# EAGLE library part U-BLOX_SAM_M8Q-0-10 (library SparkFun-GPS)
u-blox SAM-M8Q The u-blox concurrent SAM-M8Q GNSS patch antenna module benefits from the exceptional performance of the u-blox M8 multi-GNSS engine. The SAM-M8Q module offers high sensitivity and minimal acquisition times in an ultra compact form factor. The SAM-M8Q module utilizes concurrent reception of up to three GNSS systems (GPS/Galileo and GLONASS), recognizes multiple constellations simultaneously and provides outstanding positioning accuracy in scenarios where urban canyon or weak signals are involved. For even better and faster positioning improvement, the SAM-M8Q supports augmentation of QZSS, GAGAN and IMES together with WAAS, EGNOS, MSAS. The SAM-M8Q also supports message integrity protection, geofencing, and spoofing detection with configurable interface settings to easily fit to customer applications.
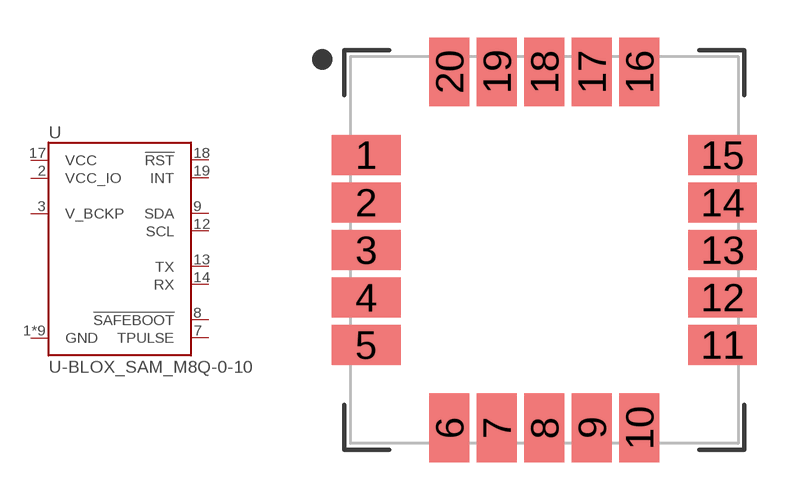
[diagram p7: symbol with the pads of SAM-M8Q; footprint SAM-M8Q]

Designator prefix U

## U-BLOX_SAM_M8Q-0-10 (PROD_ID: IC-14070)  [SAM-M8Q]
1  GND
2  VCC_IO
3  V_BCKP
4  GND
5  GND
6  GND
7  TPULSE
8  !SAFEBOOT
9  SDA
10  GND
11  GND
12  SCL
13  TX
14  RX
15  GND
16  GND
17  VCC
18  !RST
19  INT
20  GND

## Footprint SAM-M8Q (pad centres in mm)
SAM-M8Q-0-10 Physical Characteristics 15x15x6.3mm Module is a Chip Antenna/GPS Unit combined
smd 2.75 x 1.6: 1 -7.125,3.8; 2 -7.125,1.9; 3 -7.125,0; 4 -7.125,-1.9; 5 -7.125,-3.8; 11 7.125,-3.8; 12 7.125,-1.9; 13 7.125,0; 14 7.125,1.9; 15 7.125,3.8
smd 1.6 x 2.75: 6 -3.8,-7.125; 7 -1.9,-7.125; 8 0,-7.125; 9 1.9,-7.125; 10 3.8,-7.125; 16 3.8,7.125; 17 1.9,7.125; 18 0,7.125; 19 -1.9,7.125; 20 -3.8,7.125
